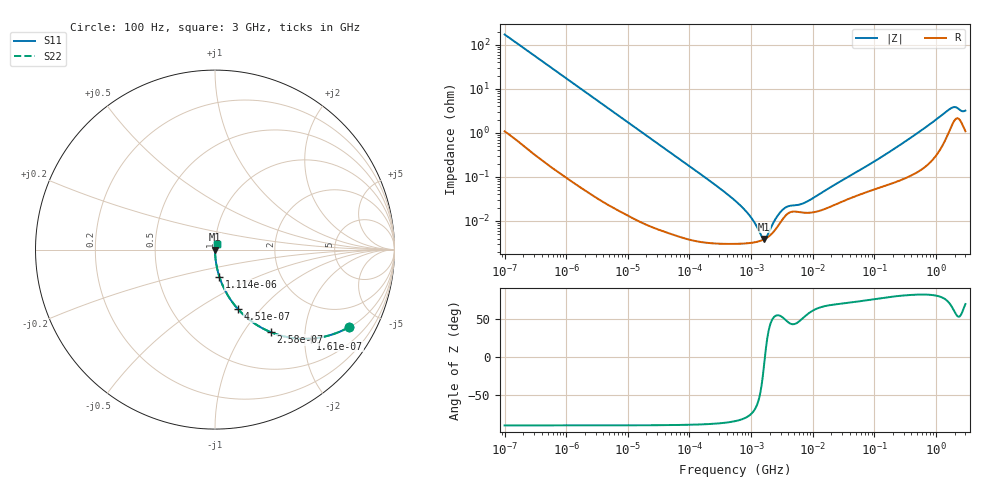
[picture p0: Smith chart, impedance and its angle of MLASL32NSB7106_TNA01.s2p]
! MLASL32NSB7106_TNA01  S-PARAMETER MODEL  ( Standard Model )
! Model Generated by TAIYO YUDEN Corporation (http://www.ty-top.com)
! Version 1.0
! TAIYO YUDEN Control No. 220601
! Copyright(c) 2009 TAIYO YUDEN CO.,LTD. All Rights Reserved.
! Product Description (link to TY-COMPAS)
! https://ds.yuden.co.jp/TYCOMPAS/or/detail?pn=MLASL32NSB7106KTNA01&u=M
! Products Name : Multilayer Ceramic Capacitors
! Characteristics :
!  Capacitance : 10 [uF] , Rated Voltage : 10 [V] , TCC : X7R
!  Case Size : 3.2 x 2.5 / 0.126 x 0.098 [mm/inch] , Thickness : 1.9 / 0.075 [mm/inch]
!  (Conditions: Temperature = 25 [degC] , DC Bias Voltage = 0 [V])
! External Node Assignments :
!  1  o---| |---o  2
! GND o---------o GND
! Frequency Range : 100Hz  -  3GHz  [ 401 STEP ]
# MHZ S RI R 50
! Freq[MHz].  S11 Real  S11 Imag  S21 Real  S21 Imag  S12 Real  S12 Imag  S22 Real  S22 Imag
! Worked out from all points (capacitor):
!   401 points, 100 Hz to 3 GHz, reference 50 ohm
!   read as one part in series: C = 9.28 uF near 109 Hz
!   lowest |Z| = 3.91 mohm at 1.607 MHz (marker M1)
!   series resonance near 1.673 MHz, so ESL is about 970 pH
!   S11 on the Smith chart (normalised r, x): 100 Hz: 1.02, -3.43; 161 Hz: 1.01, -2.14; 258 Hz: 1.01, -1.34; 451 Hz: 1.00, -0.76; 1.114 kHz: 1.00, -0.31; 3 GHz: 1.02, +0.06
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0.0001  0.7446 -0.4329  0.2554 0.4329  0.2554 0.4329  0.7446 -0.4329
0.000161  0.5335 -0.4958  0.4665 0.4958  0.4665 0.4958  0.5335 -0.4958
0.000258  0.3093 -0.4593  0.6907 0.4593  0.6907 0.4593  0.3093 -0.4593
0.000451  0.1288 -0.3323  0.8712 0.3323  0.8712 0.3323  0.1288 -0.3323
0.001114  0.0243 -0.1513  0.9757 0.1513  0.9757 0.1513  0.0243 -0.1513
0.001788  0.00983 -0.0958  0.9902 0.0958  0.9902 0.0958  0.00983 -0.0958
0.005476  0.00121 -0.0317  0.9988 0.0317  0.9988 0.0317  0.00121 -0.0317
0.031977  9.3e-05 -0.00547  0.9999 0.00547  0.9999 0.00547  9.3e-05 -0.00547
0.231582  3.17e-05 -0.000747  1 0.000747  1 0.000747  3.17e-05 -0.000747
0.547723  3.03e-05 -0.000289  1 0.000289  1 0.000289  3.03e-05 -0.000289
1.09055  3.24e-05 -9.52e-05  1 9.52e-05  1 9.52e-05  3.24e-05 -9.52e-05
1.6065  3.8e-05 -8.97e-06  1 8.97e-06  1 8.97e-06  3.8e-05 -8.97e-06
2.266852  5.5e-05 6.9e-05  0.9999 -6.9e-05  0.9999 -6.9e-05  5.5e-05 6.9e-05
3.639519  0.000133 0.000153  0.9999 -0.000153  0.9999 -0.000153  0.000133 0.000153
6.648799  0.000156 0.000188  0.9998 -0.000188  0.9998 -0.000188  0.000156 0.000188
9.794414  0.000156 0.000281  0.9998 -0.000281  0.9998 -0.000281  0.000156 0.000281
175.1444  0.00069 0.00362  0.9993 -0.00362  0.9993 -0.00362  0.00069 0.00362
559.889  0.00153 0.0109  0.9985 -0.0109  0.9985 -0.0109  0.00153 0.0109
1714.41  0.0134 0.0325  0.9866 -0.0325  0.9866 -0.0325  0.0134 0.0325
2036.508  0.0205 0.0317  0.9795 -0.0317  0.9795 -0.0317  0.0205 0.0317
2636.591  0.0167 0.0257  0.9833 -0.0257  0.9833 -0.0257  0.0167 0.0257
3000  0.0116 0.0295  0.9884 -0.0295  0.9884 -0.0295  0.0116 0.0295
